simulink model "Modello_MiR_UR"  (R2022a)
settings: Solver=FixedStepAuto  StartTime=0.0  StopTime=time_s(end,1)  FixedStep=Sim.dt*10  RelTol=1e-3  EnableMultiTasking=on
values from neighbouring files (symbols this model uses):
  a = 0.250    (= 0.25)    [Modello_MiR_UR_script.m]    (also in Modello_MiR_2ruote_script.m; Modello_MiR_6ruote_script.m; Modello_MiR_6ruote_validato_script.m)
  a1 = 0.18265    [Modello_MiR_UR_script.m]    (also in UR_DHtable_e.m = 0; Modello_MiR_2ruote_script.m = deg2rad(5); Modello_MiR_6ruote_script.m = deg2rad(5); Modello_MiR_6ruote_validato_script.m)
  a2 = 0.40857    [Modello_MiR_UR_script.m]    (also in UR_DHtable_e.m = 612; Modello_MiR_2ruote_script.m = deg2rad(25); Modello_MiR_6ruote_script.m = deg2rad(25); Modello_MiR_6ruote_validato_script.m)
  Att_C1 = 0.01    [Modello_MiR_UR_script.m]    (also in Modello_MiR_6ruote_validato_script.m)
  Att_C2 = 0.01    [Modello_MiR_UR_script.m]    (also in Modello_MiR_6ruote_validato_script.m)
  Att_C5 = 0.01    [Modello_MiR_UR_script.m]    (also in Modello_MiR_6ruote_validato_script.m)
  Att_C6 = 0.01    [Modello_MiR_UR_script.m]    (also in Modello_MiR_6ruote_validato_script.m)
  b = 0.1875    [Modello_MiR_UR_script.m]    (also in Modello_MiR_2ruote_script.m; Modello_MiR_6ruote_script.m; Modello_MiR_6ruote_validato_script.m)
  b_caster = 0.07    [Modello_MiR_UR_script.m]    (also in Modello_MiR_2ruote_script.m; Modello_MiR_6ruote_script.m; Modello_MiR_6ruote_validato_script.m)
  bd = 0.205    [Modello_MiR_UR_script.m]    (also in Modello_MiR_2ruote_script.m; Modello_MiR_6ruote_script.m; Modello_MiR_6ruote_validato_script.m)
  F23MIR = @(u) (mv*9.801/4)-(mv*h*u(5)+(mv*9.801/4)*(2*a-b_caster*(cos(u(1))+cos(u(2)))))/(4*a-b_caster*(cos(u(1))+cos(u(2)))+b_caster*(cos(u(3))+cos(u(4))))    [Modello_MiR_UR_script.m]
  F23UR5 = @(u) (u(7)/4)-u(11)    [Modello_MiR_UR_script.m]
  F43MIR = @(u) (1/(2*bd))*(mv*u(6)*h+((mv*h*u(5)+(mv*9.801/4)*(2*a-b_caster*(cos(u(1))+cos(u(2)))))/(4*a-b_caster*(cos(u(1))+cos(u(2)))+b_caster*(cos(u(3))+cos(u(4)))))*(2*bd-b_caster*(sin(u(3))+sin(u(4))))+((mv*9.801/4)-(mv*h*u(5)+(mv*9.801/4)*(2*a-b_caster*(cos(u(1))+cos(u(2)))))/(4*a-b_caster*(cos(u(1))+cos(u(2)))+b_caster*(cos(u(3))+cos(u(4)))))*(2*bd-b_caster*(sin(u(1))+sin(u(2)))))    [Modello_MiR_UR_script.m]
  F43UR5 = @(u) (1/(2*bd))*(u(8) - u(6)*H +u(11)*(2*bd-b_caster*(sin(u(3))+sin(u(4))))+u(12)*(2*bd-b_caster*(sin(u(1))+sin(u(2)))))    [Modello_MiR_UR_script.m]
  F63MIR = @(u) (mv*h*u(5)+(mv*9.801/4)*(2*a-b_caster*(cos(u(1))+cos(u(2)))))/(4*a-b_caster*(cos(u(1))+cos(u(2)))+b_caster*(cos(u(3))+cos(u(4))))    [Modello_MiR_UR_script.m]
  F63UR5 = @(u)(-a*u(7)/2 -u(5)*H -u(9) +(u(7)/4)*(2*a-b_caster*(cos(u(1))+cos(u(2)))))/(4*a-b_caster*(cos(u(1))+cos(u(2)))+b_caster*(cos(u(3))+cos(u(4))))    [Modello_MiR_UR_script.m]
  f_c = 0.29564    [Modello_MiR_UR_script.m]    (also in Modello_MiR_6ruote_validato_script.m)
  f_d3 = 0.35846    [Modello_MiR_UR_script.m]    (also in Modello_MiR_6ruote_validato_script.m)
  f_d4 = 0.2333    [Modello_MiR_UR_script.m]    (also in Modello_MiR_6ruote_validato_script.m)
  fa_c = 0.27474    [Modello_MiR_UR_script.m]    (also in Modello_MiR_6ruote_validato_script.m)
  fa_d3 = 0.3694    [Modello_MiR_UR_script.m]    (also in Modello_MiR_6ruote_validato_script.m)
  fa_d4 = 0.28065    [Modello_MiR_UR_script.m]    (also in Modello_MiR_6ruote_validato_script.m)
  fm_fun = @(u) (u <= -am2 || u >= am2) * 0 + (u > -am2 && u <= -am1) * (- u* Mza/(am2 -am1) - Mza* am2/(am2 -am1)) +           + (u > -am1 && u <= am1) * (Mza * u / am1) + (u > am1 && u < am2) * (Mza * u /(am1 -am2) - Mza * am2 /(am1 - am2))    [Modello_MiR_UR_script.m]    (also in Modello_MiR_6ruote_script.m = @(u) (u <= -am2 | u >= am2)*0 + (u > -am2 && u <= -am1)*(- u; Modello_MiR_6ruote_validato_script.m)
  Hi = 1    [UR5e_data.m]
  Icw_1 = 1/2 * mcw * rc^2    (= 0.002004225735)    [Modello_MiR_UR_script.m]    (also in Modello_MiR_2ruote_script.m; Modello_MiR_6ruote_script.m; Modello_MiR_6ruote_validato_script.m)
  Icw_2 = 1/12 * mcw * ec^2 + 1/4 * mcw * rc^2    (= 0.00104098243873)    [Modello_MiR_UR_script.m]    (also in Modello_MiR_2ruote_script.m; Modello_MiR_6ruote_script.m; Modello_MiR_6ruote_validato_script.m)
  Idw_1 = 1/2 * mdw * rd^2    (= 0.00551836278784)    [Modello_MiR_UR_script.m]    (also in Modello_MiR_2ruote_script.m; Transfer_Function_Gol_Gcl.m = Inertia_vect(jj,1); Modello_MiR_6ruote_script.m; Modello_MiR_6ruote_validato_script.m)
  iMax = 20.7*1.1    (= 22.77)    [Modello_MiR_UR_script.m]    (also in Modello_MiR_2ruote_script.m; Modello_MiR_6ruote_script.m; Modello_MiR_6ruote_validato_script.m)
  Iv = mv * (l^2 + w^2)  / 12    (= 6.75343333333)    [Modello_MiR_UR_script.m]    (also in Modello_MiR_2ruote_script.m; Modello_MiR_6ruote_script.m; Modello_MiR_6ruote_validato_script.m = 8.95033333333)
  Kc = 0.15    [Modello_MiR_UR_script.m]    (also in Modello_MiR_2ruote_script.m; Modello_MiR_6ruote_script.m; Modello_MiR_6ruote_validato_script.m)
  Ki_i = 1    [Modello_MiR_UR_script.m]    (also in Modello_MiR_2ruote_script.m; Modello_MiR_6ruote_script.m; Modello_MiR_6ruote_validato_script.m)
  Ki_v = 1    [Modello_MiR_UR_script.m]    (also in Modello_MiR_2ruote_script.m; Modello_MiR_6ruote_script.m; Modello_MiR_6ruote_validato_script.m)
  kk = 0.00005    (= 5e-05)    [Modello_MiR_UR_script.m]    (also in Modello_MiR_2ruote_script.m; Modello_MiR_6ruote_script.m; Modello_MiR_6ruote_validato_script.m)
  Kp_i = 5    [Modello_MiR_UR_script.m]    (also in Modello_MiR_2ruote_script.m; Modello_MiR_6ruote_script.m; Modello_MiR_6ruote_validato_script.m)
  Kp_v = 5    [Modello_MiR_UR_script.m]    (also in Modello_MiR_2ruote_script.m; Modello_MiR_6ruote_script.m; Modello_MiR_6ruote_validato_script.m)
  kv = 1.5e-6    (= 1.5e-06)    [Modello_MiR_UR_script.m]    (also in Modello_MiR_2ruote_script.m; Modello_MiR_6ruote_script.m; Modello_MiR_6ruote_validato_script.m)
  L = R * tauE    (= 0.00181134822805)    [Modello_MiR_UR_script.m]    (also in Modello_MiR_2ruote_script.m; Modello_MiR_6ruote_script.m; Modello_MiR_6ruote_validato_script.m)
  mcw = rc^2 * pi * ec * rhopoliu + 1    (= 1.02616357632)    [Modello_MiR_UR_script.m]    (also in Modello_MiR_2ruote_script.m; Modello_MiR_6ruote_script.m; Modello_MiR_6ruote_validato_script.m)
  mv = 83    [Modello_MiR_UR_script.m]    (also in Modello_MiR_2ruote_script.m; Modello_MiR_6ruote_script.m; Modello_MiR_6ruote_validato_script.m = 110)
  Phi1_start = psi_mir(1,1)    [Modello_MiR_UR_script.m]    (also in Modello_MiR_6ruote_validato_script.m)
  Phi2_start = psi_mir(1,1)    [Modello_MiR_UR_script.m]    (also in Modello_MiR_6ruote_validato_script.m)
  Phi5_start = psi_mir(1,1)    [Modello_MiR_UR_script.m]    (also in Modello_MiR_6ruote_validato_script.m)
  Phi6_start = psi_mir(1,1)    [Modello_MiR_UR_script.m]    (also in Modello_MiR_6ruote_validato_script.m)
  Psi_start = psi_mir(1,1)    [Modello_MiR_UR_script.m]    (also in Modello_MiR_6ruote_script.m = 1.57079632679; Modello_MiR_6ruote_validato_script.m)
  q0 = [qset.q1.signals.values(1),qset.q2.signals.values(1),qset.q3.signals.values(1),qset.q4.signals.values(1),qset.q5.signals.values(1),qset.q6.signals.values(1)]    [UR5e_simmot.m]
  R = velMax * TorqueMax / (iMax)^2    (= 1.81134822805)    [Modello_MiR_UR_script.m]    (also in Modello_MiR_2ruote_script.m; Modello_MiR_6ruote_script.m; Modello_MiR_6ruote_validato_script.m)
  rap_rid = 10.167    [Modello_MiR_UR_script.m]    (also in Modello_MiR_2ruote_script.m; Modello_MiR_6ruote_script.m; Modello_MiR_6ruote_validato_script.m)
  rc = 0.125/2    (= 0.0625)    [Modello_MiR_UR_script.m]    (also in Modello_MiR_2ruote_script.m; Modello_MiR_6ruote_script.m; Modello_MiR_6ruote_validato_script.m)
  rd = 0.1    [Modello_MiR_UR_script.m]    (also in Modello_MiR_2ruote_script.m; Modello_MiR_6ruote_script.m; Modello_MiR_6ruote_validato_script.m)
  s = 1i*s    [Transfer_Function_Gol_Gcl.m]
  s1 = 0.18987    [Modello_MiR_UR_script.m]    (also in Modello_MiR_2ruote_script.m = 0.2; Modello_MiR_6ruote_script.m = 0.2; Modello_MiR_6ruote_validato_script.m)
  s2 = 0.99533    [Modello_MiR_UR_script.m]    (also in Modello_MiR_2ruote_script.m = 0.8; Modello_MiR_6ruote_script.m = 0.8; Modello_MiR_6ruote_validato_script.m)
  Sx = spline(x ,fl_fun(x),zx)    [Modello_MiR_6ruote_script.m]
  Sy = spline(x ,ft_fun(x),zy)    [Modello_MiR_6ruote_script.m]
  tau_i = 1/(2000*2*pi)    (= 7.95774715459e-05)    [UR5e_data.m]    (also in Transfer_Function_Gol_Gcl.m = Kp_i/Ki_i)
  VaMax = Kc * velMax    (= 41.2443991527)    [Modello_MiR_UR_script.m]    (also in Modello_MiR_2ruote_script.m; Modello_MiR_6ruote_script.m; Modello_MiR_6ruote_validato_script.m)
  X_start = traj(1,1)    [Modello_MiR_UR_script.m]    (also in Modello_MiR_2ruote_script.m = input('Inserire coordinata x iniziale'); Modello_MiR_6ruote_script.m = input('Inserire coordinata x iniziale'); Modello_MiR_6ruote_validato_script.m)
  Y_start = traj(1,2)    [Modello_MiR_UR_script.m]    (also in Modello_MiR_2ruote_script.m = input('Inserire coordinata y iniziale'); Modello_MiR_6ruote_script.m = input('Inserire coordinata y iniziale'); Modello_MiR_6ruote_validato_script.m)
undefined symbols (not defined in the file or in its folder): deg, Driver1, Driver2, Driver3, Driver4, Driver5, Driver6, Ground, J1, J2, J3, J4, J5, J6, kg, L1, L2, L3, L4, L5, L6, m, Motor, N, X, Y, z, Z
libraries: sm_lib x33, nesl_utility x30, slpidlib x10
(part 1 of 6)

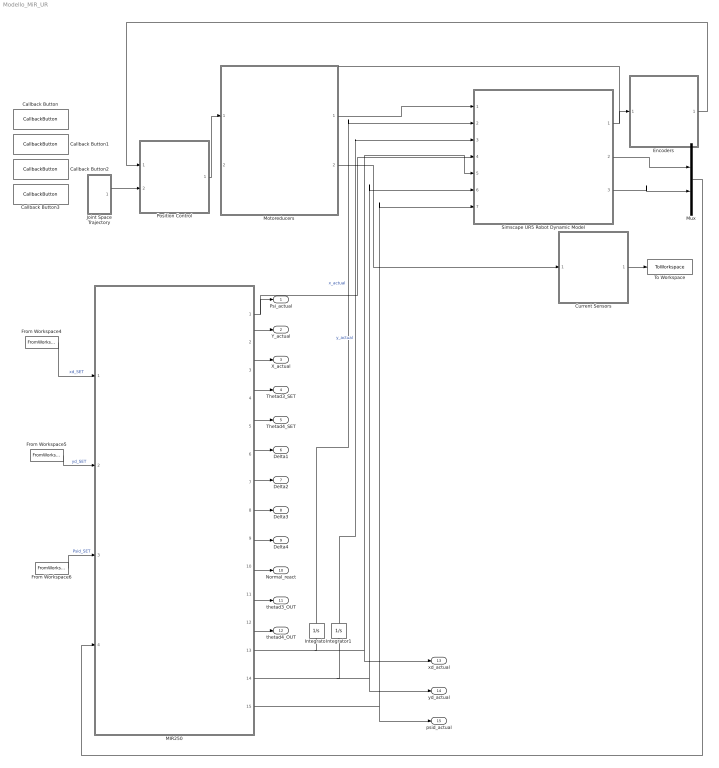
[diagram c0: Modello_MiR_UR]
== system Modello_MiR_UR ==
  Callback Button : CallbackButton  ButtonText=Reset
  Callback Button1 : CallbackButton  ButtonText=Parameters Setting
  Callback Button2 : CallbackButton  ButtonText=Motion Setting
  Callback Button3 : CallbackButton  ButtonText=Current Plotting
  Current Sensors : Subsystem
  Encoders : Subsystem
  From Workspace4 : FromWorkspace  VariableName=[time_v xd_set]
  From Workspace5 : FromWorkspace  VariableName=[time_v yd_set]
  From Workspace6 : FromWorkspace  VariableName=[ time_v psid_set]
  Integrator : Integrator
  Integrator1 : Integrator
  Joint Space Trajectory : Subsystem
  MIR250 : Subsystem
  Motoreducers : Subsystem
  Mux : Mux  Inputs=2
  Position Control : Subsystem
  Simscape UR5 Robot Dynamic Model : Subsystem
  To Workspace : ToWorkspace  VariableName=iFB  SaveFormat=Timeseries  SampleTime=-1
  Psi_actual : Outport
  Y_actual : Outport  Port=2
  X_actual : Outport  Port=3
  Thetad3_SET : Outport  Port=4
  Thetad4_SET : Outport  Port=5
  Delta1 : Outport  Port=6
  Delta2 : Outport  Port=7
  Delta3 : Outport  Port=8
  Delta4 : Outport  Port=9
  Normal_react : Outport  Port=10
  thetad3_OUT : Outport  Port=11
  thetad4_OUT : Outport  Port=12
  xd_actual : Outport  Port=13
  yd_actual : Outport  Port=14
  psid_actual : Outport  Port=15
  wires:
  Encoders/1(qFB,qdFB,qddFB) -> Position Control/1(qFB,qdFB,qddFB)
  Position Control/1(Vset) -> Motoreducers/1(Vset)
  Simscape UR5 Robot Dynamic Model/1(q,qd,qdd) -> Encoders/1(q,qd,qdd), Motoreducers/2(q,qd,qdd)
  Motoreducers/1(Tu) -> Simscape UR5 Robot Dynamic Model/1(T)
  Motoreducers/2(i) -> Current Sensors/1(i)
  Current Sensors/1(iFB) -> To Workspace/1
  Joint Space Trajectory/1(qset) -> Position Control/2(qset,qdset,qddset)
  From Workspace4/1 -> MIR250/1(xd_set)  "xd_SET"
  From Workspace5/1 -> MIR250/2(yd_set)  "yd_SET"
  From Workspace6/1 -> MIR250/3(Psid_set)  "Psid_SET"
  Simscape UR5 Robot Dynamic Model/2(Force constrain) -> Mux/1
  Simscape UR5 Robot Dynamic Model/3(Torque constrain) -> Mux/2
  MIR250/1(Psi_actual) -> Simscape UR5 Robot Dynamic Model/4(psi_actual), Psi_actual/1
  MIR250/2(Y_actual) -> Y_actual/1
  MIR250/3(X_actual) -> X_actual/1
  MIR250/4(Thetad3_SET) -> Thetad3_SET/1
  MIR250/5(Thetad4 SET) -> Thetad4_SET/1
  MIR250/6(Delta1) -> Delta1/1
  MIR250/7(Delta2) -> Delta2/1
  MIR250/8(Delta3) -> Delta3/1
  MIR250/9(Delta4) -> Delta4/1
  MIR250/10(Normal_react) -> Normal_react/1
  MIR250/11(thetad3_OUT) -> thetad3_OUT/1
  MIR250/12(Thetad4_OUT) -> thetad4_OUT/1
  Mux/1 -> MIR250/4(UR5_forces)
  Integrator/1 -> Simscape UR5 Robot Dynamic Model/2(x_actual)  "x_actual"
  Integrator1/1 -> Simscape UR5 Robot Dynamic Model/3(y_actual)  "y_actual"
  MIR250/13(xd_actual) -> xd_actual/1, Simscape UR5 Robot Dynamic Model/5(xd_actual), Integrator/1
  MIR250/14(yd_actual) -> Simscape UR5 Robot Dynamic Model/6(yd_actual), yd_actual/1, Integrator1/1
  MIR250/15(Psid_actual) -> psid_actual/1, Simscape UR5 Robot Dynamic Model/7(psid_actual)

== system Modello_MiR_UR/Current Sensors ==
  i : Inport
  Demux1 : Demux  Outputs=6
  Mux1 : Mux  Inputs=6
  Subsystem : Subsystem
  iFB : Outport
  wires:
  Subsystem/1(i1FB) -> Mux1/1
  Demux1/4 -> Subsystem/4(i5)
  Demux1/5 -> Subsystem/5(i3)
  Subsystem/6(i6FB) -> Mux1/6
  Demux1/2 -> Subsystem/2(i4)
  Subsystem/3(i2FB) -> Mux1/3
  Demux1/6 -> Subsystem/6(i6)
  Demux1/3 -> Subsystem/3(i2)
  Demux1/1 -> Subsystem/1(i1)
  Subsystem/4(i5FB) -> Mux1/4
  Subsystem/2(i4FB) -> Mux1/2
  Subsystem/5(i3FB) -> Mux1/5
  Mux1/1 -> iFB/1
  i/1 -> Demux1/1

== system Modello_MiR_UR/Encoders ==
  q,qd,qdd : Inport
  Demux1 : Demux  Outputs=6
  Mux1 : Mux  Inputs=6
  Subsystem : Subsystem
  qFB,qdFB,qddFB : Outport
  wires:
  q,qd,qdd/1 -> Demux1/1
  Mux1/1 -> qFB,qdFB,qddFB/1
  Subsystem/5(q5FB,qd5FB,qdd5FB) -> Mux1/5
  Subsystem/2(q2FB,qd2FB,qdd2FB) -> Mux1/2
  Subsystem/4(q4FB,qd4FB,qdd4FB) -> Mux1/4
  Demux1/1 -> Subsystem/1(q1,qd1,qdd2)
  Demux1/3 -> Subsystem/3(q3,qd3,qdd3)
  Demux1/6 -> Subsystem/6(q6,qd6,qdd6)
  Subsystem/3(q3FB,qd3FB,qdd3FB) -> Mux1/3
  Demux1/2 -> Subsystem/2(q2,qd2,qdd2)
  Subsystem/6(q6FB,qd6FB,qdd6FB) -> Mux1/6
  Demux1/5 -> Subsystem/5(q5,qd5,qdd5)
  Demux1/4 -> Subsystem/4(q4,qd4,qdd4)
  Subsystem/1(q1FB,qd1FB,qdd1FB) -> Mux1/1

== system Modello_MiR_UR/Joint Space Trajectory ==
  From Workspace : FromWorkspace  VariableName=qset.q1
  From Workspace1 : FromWorkspace  VariableName=qset.q2
  From Workspace2 : FromWorkspace  VariableName=qset.q3
  From Workspace3 : FromWorkspace  VariableName=qset.q4
  From Workspace4 : FromWorkspace  VariableName=qset.q5
  From Workspace5 : FromWorkspace  VariableName=qset.q6
  Mux2 : Mux  Inputs=6
  qset : Outport
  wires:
  From Workspace2/1 -> Mux2/3
  From Workspace/1 -> Mux2/1
  From Workspace3/1 -> Mux2/4
  From Workspace4/1 -> Mux2/5
  From Workspace5/1 -> Mux2/6
  From Workspace1/1 -> Mux2/2
  Mux2/1 -> qset/1

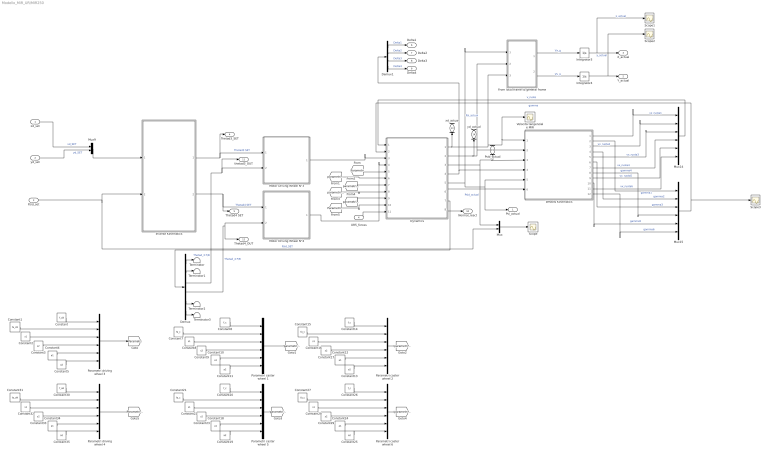
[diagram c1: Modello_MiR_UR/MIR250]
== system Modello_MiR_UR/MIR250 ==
  xd_set : Inport
  yd_set : Inport  Port=2
  Psid_set : Inport  Port=3
  UR5_forces : Inport  Port=4
  " Wheels Kinematics" : Subsystem
  Constant : Constant  Value=f_d3
  Constant1 : Constant  Value=fa_d3
  Constant{4,10,12,18,24,34} (6 alike) : Constant  Value=a1
  Constant{5,11,13,19,25,35} (6 alike) : Constant  Value=a2
  Constant{6,14,20,26} (4 alike) : Constant  Value=f_c
  Constant{7,15,21,27} (4 alike) : Constant  Value=fa_c
  Constant{2,8,16,22,28,32} (6 alike) : Constant  Value=s1
  Constant{3,9,17,23,29,33} (6 alike) : Constant  Value=s2
  Constant30 : Constant  Value=f_d4
  Constant31 : Constant  Value=fa_d4
  Demux : Demux  Outputs=6
  Demux1 : Demux
  Dynamics : Subsystem
  From local frame to general frame : Subsystem
  Integrator3 : Integrator  InitialCondition=X_start
  Integrator4 : Integrator  InitialCondition=Y_start
  Inverse Kinematics : Subsystem
  Motor Driving Wheel N°3 : Subsystem
  Motor Driving Wheel N°4 : Subsystem
  Mux : Mux  Inputs=2
  Mux14 : Mux  Inputs=6
  Mux15 : Mux  Inputs=6
  Mux9 : Mux  Inputs=2
  Parametri caster wheel {1..2,5..6} (4 alike) : Mux  Inputs=6
  Parametri driving wheel 3 : Mux  Inputs=6
  Parametri driving wheel 4 : Mux  Inputs=6
  Scope{,1..3} (4 alike) : Scope
  Terminator{,1..3} (4 alike) : Terminator
  Velocità tangenziale MIR : Scope
  Psi_actual : Outport
  Y_actual : Outport  Port=2
  X_actual : Outport  Port=3
  Thetad3_SET : Outport  Port=4
  Thetad4 SET : Outport  Port=5
  Delta1 : Outport  Port=6
  Delta2 : Outport  Port=7
  Delta3 : Outport  Port=8
  Delta4 : Outport  Port=9
  Normal_react : Outport  Port=10
  thetad3_OUT : Outport  Port=11
  Thetad4_OUT : Outport  Port=12
  xd_actual : Outport  Port=13
  yd_actual : Outport  Port=14
  Psid_actual : Outport  Port=15
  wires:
  Demux1/4 -> Delta4/1  "Delta4"
  Constant5/1 -> Parametri driving wheel 3/6
  [Parametri] -> Dynamics/5(parametri_dw3)
  Demux1/1 -> Delta1/1  "Delta1"
  Mux/1 -> Scope/1
  Motor Driving Wheel N°4/1(Cm_R) -> Dynamics/4(Cm4)
  " Wheels Kinematics"/1(vx_ruota1) -> Mux14/1  "vx_ruota1"
  Mux14/1 -> Dynamics/1(vx_ruote)  "v_ruote"
  From local frame to general frame/1(Vx_g) -> Integrator3/1  "Vx_g"
  Dynamics/2(yd) -> yd_actual/1, From local frame to general frame/2(Vy), " Wheels Kinematics"/2(yd)
  Demux/2 -> Terminator1/1
  Demux/4 -> Thetad4_OUT/1, Motor Driving Wheel N°4/2(ThetadR_FB)  "Thetad_4 F/B"
  Integrator3/1 -> Scope1/1, X_actual/1  "x_actual"
  " Wheels Kinematics"/6(gamma3) -> Mux15/3  "gamma3"
  Mux9/1 -> Inverse Kinematics/1(vSet)
  Integrator4/1 -> Scope2/1, Y_actual/1  "y_actual"
  Dynamics/3(Psid) -> Psid_actual/1, " Wheels Kinematics"/3(Psid), Mux/1  "Psid_actual"
  Demux/5 -> Terminator2/1
  " Wheels Kinematics"/5(vx_ruota3) -> Mux14/3  "vx_ruota3"
  Dynamics/7(Thetad) -> Demux/1
  Demux/6 -> Terminator3/1
  Dynamics/5(Psi) -> From local frame to general frame/1(Psi), Psi_actual/1, " Wheels Kinematics"/5(Psi)  "Psi_actual"
  " Wheels Kinematics"/3(vx_ruota2) -> Mux14/2  "vx_ruota2"
  " Wheels Kinematics"/8(gamma4) -> Mux15/4  "gamma4"
  " Wheels Kinematics"/7(vx_ruota4) -> Mux14/4  "vx_ruota4"
  Dynamics/4(Delta) -> Demux1/1, " Wheels Kinematics"/4(Delta)
  From local frame to general frame/2(Vy_g) -> Integrator4/1  "Vy_g"
  " Wheels Kinematics"/12(gamma6) -> Mux15/6  "gamma6"
  " Wheels Kinematics"/4(gamma2) -> Mux15/2  "gamma2"
  Constant20/1 -> Parametri caster wheel 5/1
  Parametri caster wheel 6/1 -> [parametri_cw6]
  yd_set/1 -> Mux9/2  "yd_SET"
  Demux1/2 -> Delta2/1  "Delta2"
  Constant27/1 -> Parametri caster wheel 6/2
  Constant21/1 -> Parametri caster wheel 5/2
  [parametri_cw5] -> Dynamics/8(parametri_cw5)
  " Wheels Kinematics"/9(vx_ruota5) -> Mux14/5  "vx_ruota5"
  Constant26/1 -> Parametri caster wheel 6/1
  Constant24/1 -> Parametri caster wheel 6/5
  Motor Driving Wheel N°3/1(Cm_L) -> Dynamics/3(Cm3)
  [parametri_cw2] -> Dynamics/7(parametri_cw2)
  Constant28/1 -> Parametri caster wheel 6/3
  Parametri caster wheel 1/1 -> [parametri_cw1]
  Constant29/1 -> Parametri caster wheel 6/4
  Constant6/1 -> Parametri caster wheel 1/1
  Inverse Kinematics/2(ThetaDotR) -> Thetad4 SET/1, Motor Driving Wheel N°4/1(ThetadR_SET)  "Thetad4 SET"
  Constant15/1 -> Parametri caster wheel 2/2
  Parametri driving wheel 3/1 -> [Parametri]
  Constant4/1 -> Parametri driving wheel 3/5
  Parametri caster wheel 2/1 -> [parametri_cw2]
  Constant12/1 -> Parametri caster wheel 2/5
  Constant7/1 -> Parametri caster wheel 1/2
  Dynamics/6(Phid) -> " Wheels Kinematics"/6(Phid)
  Psid_set/1 -> Mux/2, Inverse Kinematics/2(psiDotSet)  "Psid_SET"
  xd_set/1 -> Mux9/1  "xd_SET"
  Constant10/1 -> Parametri caster wheel 1/5
  Mux15/1 -> Scope3/1, Dynamics/2(gamma)  "gamma"
  Constant2/1 -> Parametri driving wheel 3/3
  Constant1/1 -> Parametri driving wheel 3/2
  Dynamics/8(Normal_react) -> Normal_react/1
  Demux/1 -> Terminator/1
  Constant18/1 -> Parametri caster wheel 5/5
  " Wheels Kinematics"/2(gamma1) -> Mux15/1  "gamma1"
  Constant8/1 -> Parametri caster wheel 1/3
  Inverse Kinematics/1(ThetaDotL) -> Thetad3_SET/1, Motor Driving Wheel N°3/1(ThetadL_SET)  "Thetad3 SET"
  Constant17/1 -> Parametri caster wheel 2/4
  Constant16/1 -> Parametri caster wheel 2/3
  Constant30/1 -> Parametri driving wheel 4/1
  Parametri driving wheel 4/1 -> [Parametri_dw4]
  Demux/3 -> thetad3_OUT/1, Motor Driving Wheel N°3/2(ThetadL_FB)  "Thetad_3 F/B"
  [Parametri_dw4] -> Dynamics/10(parametri_dw4)
  Constant3/1 -> Parametri driving wheel 3/4
  Constant22/1 -> Parametri caster wheel 5/3
  " Wheels Kinematics"/11(vx_ruota6) -> Mux14/6  "vx_ruota6"
  " Wheels Kinematics"/10(gamma5) -> Mux15/5  "gamma5"
  Constant34/1 -> Parametri driving wheel 4/5
  Constant31/1 -> Parametri driving wheel 4/2
  Constant9/1 -> Parametri caster wheel 1/4
  Constant32/1 -> Parametri driving wheel 4/3
  Constant11/1 -> Parametri caster wheel 1/6
  [parametri_cw1] -> Dynamics/6(parametri_cw1)
  Dynamics/1(xd) -> xd_actual/1, From local frame to general frame/3(Vx), Velocità tangenziale MIR/1, " Wheels Kinematics"/1(xd)
  Parametri caster wheel 5/1 -> [parametri_cw5]
  Demux1/3 -> Delta3/1  "Delta3"
  Constant33/1 -> Parametri driving wheel 4/4
  Constant14/1 -> Parametri caster wheel 2/1
  Constant19/1 -> Parametri caster wheel 5/6
  Constant13/1 -> Parametri caster wheel 2/6
  [parametri_cw6] -> Dynamics/9(parametri_cw6)
  Constant25/1 -> Parametri caster wheel 6/6
  Constant23/1 -> Parametri caster wheel 5/4
  Constant35/1 -> Parametri driving wheel 4/6
  Constant/1 -> Parametri driving wheel 3/1
  UR5_forces/1 -> Dynamics/11(UR5_forces)

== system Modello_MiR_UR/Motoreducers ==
  Vset : Inport
  q,qd,qdd : Inport  Port=2
  Demux1 : Demux  Outputs=6
  Demux2 : Demux  Outputs=6
  Mux1 : Mux  Inputs=6
  Mux2 : Mux  Inputs=6
  Subsystem : Subsystem
  Tu : Outport
  i : Outport  Port=2
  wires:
  Vset/1 -> Demux1/1
  Mux1/1 -> Tu/1
  Subsystem/5(Tu5) -> Mux1/5
  Subsystem/2(Tu2) -> Mux1/2
  Subsystem/4(Tu4) -> Mux1/4
  Demux1/1 -> Subsystem/1(Vset1)
  Demux1/3 -> Subsystem/3(Vset3)
  Demux1/6 -> Subsystem/6(Vset6)
  Subsystem/3(Tu3) -> Mux1/3
  Demux1/2 -> Subsystem/2(Vset2)
  Subsystem/6(Tu6) -> Mux1/6
  Demux1/5 -> Subsystem/5(Vset5)
  Demux1/4 -> Subsystem/4(Vset4)
  Subsystem/1(Tu1) -> Mux1/1
  Demux2/1 -> Subsystem/7(q1,qd1,qdd1)
  Demux2/2 -> Subsystem/8(q2,qd2,qdd2)
  Demux2/3 -> Subsystem/9(q3,qd3,qdd3)
  Demux2/4 -> Subsystem/10(q4,qd4,qdd4)
  Demux2/5 -> Subsystem/11(q5,qd5,qdd5)
  Demux2/6 -> Subsystem/12(q6,qd6,qdd6)
  q,qd,qdd/1 -> Demux2/1
  Subsystem/7(i1) -> Mux2/1
  Subsystem/8(i2) -> Mux2/2
  Subsystem/9(i3) -> Mux2/3
  Subsystem/10(i4) -> Mux2/4
  Subsystem/11(i5) -> Mux2/5
  Subsystem/12(i6) -> Mux2/6
  Mux2/1 -> i/1

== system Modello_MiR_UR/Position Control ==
  qFB,qdFB,qddFB : Inport
  qset,qdset,qddset : Inport  Port=2
  Demux : Demux  Outputs=6
  Demux1 : Demux  Outputs=6
  Mux : Mux  Inputs=6
  Subsystem : Subsystem
  Vset : Outport
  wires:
  Demux/1 -> Subsystem/1(q1set,qd1set,qdd1set)
  Demux/4 -> Subsystem/4(q4set,qd4set,qdd4set)
  Demux/3 -> Subsystem/3(q3set,qd3set,qdd3set)
  Demux1/1 -> Subsystem/7(q1FB,qd1FB,qdd1FB)
  Demux/5 -> Subsystem/5(q5set,qd5set,qdd5set)
  Demux1/2 -> Subsystem/8(q2FB,qd2FB,qdd2FB)
  Demux/2 -> Subsystem/2(q2set,qd2set,qdd2set)
  Demux/6 -> Subsystem/6(q6set,qd6set,qdd6set)
  Demux1/3 -> Subsystem/9(q3FB,qd3FB,qdd3FB)
  Demux1/5 -> Subsystem/11(q5FB,qd5FB,qdd5FB)
  Demux1/6 -> Subsystem/12(q6FB,qd6FB,qdd6FB)
  Subsystem/4(Vset4) -> Mux/4
  Demux1/4 -> Subsystem/10(q4FB,qd4FB,qdd4FB)
  Subsystem/2(Vset2) -> Mux/2
  Subsystem/1(Vset1) -> Mux/1
  Subsystem/5(Vset5) -> Mux/5
  Subsystem/6(Vset6) -> Mux/6
  Subsystem/3(Vset3) -> Mux/3
  qFB,qdFB,qddFB/1 -> Demux1/1
  Mux/1 -> Vset/1
  qset,qdset,qddset/1 -> Demux/1

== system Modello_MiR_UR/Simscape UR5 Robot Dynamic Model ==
  T : Inport
  x_actual : Inport  Port=2
  y_actual : Inport  Port=3
  psi_actual : Inport  Port=4
  xd_actual : Inport  Port=5
  yd_actual : Inport  Port=6
  psid_actual : Inport  Port=7
  Demux1 : Demux  Outputs=6
  Mux1 : Mux  Inputs=6
  Sinscape UR5 Robot Dynamic Model1 : Subsystem
  q,qd,qdd : Outport
  Force constrain : Outport  Port=2
  Torque constrain : Outport  Port=3
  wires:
  Sinscape UR5 Robot Dynamic Model1/1(q1,qd1,qdd1) -> Mux1/1
  Demux1/4 -> Sinscape UR5 Robot Dynamic Model1/4(T4)
  Demux1/5 -> Sinscape UR5 Robot Dynamic Model1/5(T5)
  Sinscape UR5 Robot Dynamic Model1/6(q6,qd6,qdd6) -> Mux1/6
  Demux1/2 -> Sinscape UR5 Robot Dynamic Model1/2(T2)
  Sinscape UR5 Robot Dynamic Model1/3(q3,qd3,qdd3) -> Mux1/3
  Demux1/6 -> Sinscape UR5 Robot Dynamic Model1/6(T6)
  Demux1/3 -> Sinscape UR5 Robot Dynamic Model1/3(T3)
  Demux1/1 -> Sinscape UR5 Robot Dynamic Model1/1(T1)
  Sinscape UR5 Robot Dynamic Model1/4(q4,qd4,qdd4) -> Mux1/4
  Sinscape UR5 Robot Dynamic Model1/2(q2,qd2,qdd2) -> Mux1/2
  Sinscape UR5 Robot Dynamic Model1/5(q5,qd5,qdd5) -> Mux1/5
  Mux1/1 -> q,qd,qdd/1
  T/1 -> Demux1/1
  x_actual/1 -> Sinscape UR5 Robot Dynamic Model1/7(x_actual)
  y_actual/1 -> Sinscape UR5 Robot Dynamic Model1/8(y_actual)
  psi_actual/1 -> Sinscape UR5 Robot Dynamic Model1/9(psi_actual)
  Sinscape UR5 Robot Dynamic Model1/7(Force constrain) -> Force constrain/1
  Sinscape UR5 Robot Dynamic Model1/8(Torque constrain) -> Torque constrain/1
  xd_actual/1 -> Sinscape UR5 Robot Dynamic Model1/10(xd_actual)
  yd_actual/1 -> Sinscape UR5 Robot Dynamic Model1/11(yd_actual)
  psid_actual/1 -> Sinscape UR5 Robot Dynamic Model1/12(psid_actual)

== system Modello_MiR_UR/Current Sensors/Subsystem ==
  i1 : Inport
  i4 : Inport  Port=2
  i2 : Inport  Port=3
  i5 : Inport  Port=4
  i3 : Inport  Port=5
  i6 : Inport  Port=6
  Current Sensor{1..6} (6 alike) : TransferFcn  Numerator=[Hi]  Denominator=[tau_i 1]
  i1FB : Outport
  i4FB : Outport  Port=2
  i2FB : Outport  Port=3
  i5FB : Outport  Port=4
  i3FB : Outport  Port=5
  i6FB : Outport  Port=6
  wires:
  i6/1 -> Current Sensor6/1
  i2/1 -> Current Sensor2/1
  Current Sensor2/1 -> i2FB/1
  i1/1 -> Current Sensor1/1
  Current Sensor3/1 -> i3FB/1
  Current Sensor6/1 -> i6FB/1
  i3/1 -> Current Sensor3/1
  i4/1 -> Current Sensor4/1
  Current Sensor1/1 -> i1FB/1
  Current Sensor4/1 -> i4FB/1
  i5/1 -> Current Sensor5/1
  Current Sensor5/1 -> i5FB/1

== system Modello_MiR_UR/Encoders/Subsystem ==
  q1,qd1,qdd2 : Inport
  q2,qd2,qdd2 : Inport  Port=2
  q3,qd3,qdd3 : Inport  Port=3
  q4,qd4,qdd4 : Inport  Port=4
  q5,qd5,qdd5 : Inport  Port=5
  q6,qd6,qdd6 : Inport  Port=6
  Gain{,1..5} (6 alike) : Gain
  q1FB,qd1FB,qdd1FB : Outport
  q2FB,qd2FB,qdd2FB : Outport  Port=2
  q3FB,qd3FB,qdd3FB : Outport  Port=3
  q4FB,qd4FB,qdd4FB : Outport  Port=4
  q5FB,qd5FB,qdd5FB : Outport  Port=5
  q6FB,qd6FB,qdd6FB : Outport  Port=6
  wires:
  q2,qd2,qdd2/1 -> Gain1/1
  Gain3/1 -> q4FB,qd4FB,qdd4FB/1
  Gain/1 -> q1FB,qd1FB,qdd1FB/1
  Gain1/1 -> q2FB,qd2FB,qdd2FB/1
  q4,qd4,qdd4/1 -> Gain3/1
  q3,qd3,qdd3/1 -> Gain2/1
  Gain5/1 -> q6FB,qd6FB,qdd6FB/1
  Gain2/1 -> q3FB,qd3FB,qdd3FB/1
  Gain4/1 -> q5FB,qd5FB,qdd5FB/1
  q1,qd1,qdd2/1 -> Gain/1
  q5,qd5,qdd5/1 -> Gain4/1
  q6,qd6,qdd6/1 -> Gain5/1

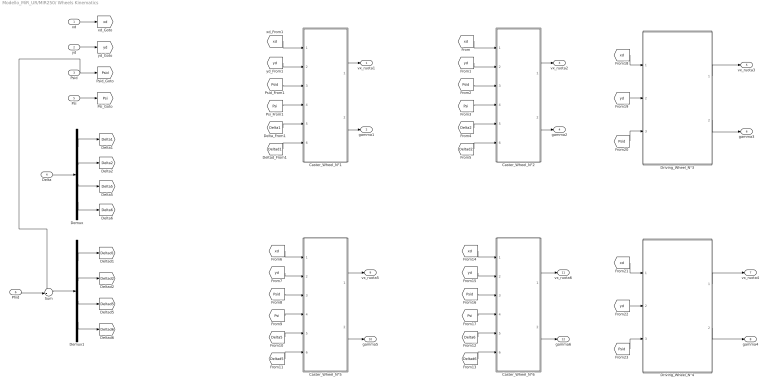
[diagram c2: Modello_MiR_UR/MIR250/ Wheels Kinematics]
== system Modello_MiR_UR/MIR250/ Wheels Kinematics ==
  xd : Inport
  yd : Inport  Port=2
  Psid : Inport  Port=3
  Delta : Inport  Port=4
  Psi : Inport  Port=5
  Phid : Inport  Port=6
  Caster_Wheel_N°1 : Subsystem
  Caster_Wheel_N°2 : Subsystem
  Caster_Wheel_N°5 : Subsystem
  Caster_Wheel_N°6 : Subsystem
  Demux : Demux
  Demux1 : Demux
  Driving_Wheel_N°3 : Subsystem
  Driving_Wheel_N°4 : Subsystem
  Sum : Sum  Inputs=-+|
  vx_ruota1 : Outport
  gamma1 : Outport  Port=2  PortDimensions=1
  vx_ruota2 : Outport  Port=3
  gamma2 : Outport  Port=4  PortDimensions=1
  vx_ruota3 : Outport  Port=5
  gamma3 : Outport  Port=6  PortDimensions=1
  vx_ruota4 : Outport  Port=7
  gamma4 : Outport  Port=8  PortDimensions=1
  vx_ruota5 : Outport  Port=9
  gamma5 : Outport  Port=10  PortDimensions=1
  vx_ruota6 : Outport  Port=11
  gamma6 : Outport  Port=12  PortDimensions=1
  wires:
  xd/1 -> [xd]
  yd/1 -> [yd]
  Psid/1 -> [Psid], Sum/1
  Delta/1 -> Demux/1
  Demux/1 -> [Delta1]
  Demux/2 -> [Delta2]
  Demux/3 -> [Delta5]
  Demux/4 -> [Delta6]
  Psi/1 -> [Psi]
  Phid/1 -> Sum/2
  Demux1/1 -> [Deltad1]
  Demux1/2 -> [Deltad2]
  Demux1/3 -> [Deltad5]
  Demux1/4 -> [Deltad6]
  [xd] -> Caster_Wheel_N°1/1(xd_From1)
  [yd] -> Caster_Wheel_N°1/2(yd_From1)
  [Psid] -> Caster_Wheel_N°1/3(Psid_From1)
  [Psi] -> Caster_Wheel_N°1/4(Psi_From1)
  [Delta1] -> Caster_Wheel_N°1/5(Delta_From1)
  [Deltad1] -> Caster_Wheel_N°1/6(Deltad_From1)
  Caster_Wheel_N°1/1(vx_ruota1) -> vx_ruota1/1
  Caster_Wheel_N°1/2(gamma1) -> gamma1/1
  [yd] -> Caster_Wheel_N°2/2(yd_From1)
  [Psi] -> Caster_Wheel_N°2/4(Psi_From1)
  [Psid] -> Caster_Wheel_N°2/3(Psid_From1)
  [xd] -> Caster_Wheel_N°2/1(xd_From1)
  [Deltad2] -> Caster_Wheel_N°2/6(Deltad_From2)
  Caster_Wheel_N°2/2(gamma2) -> gamma2/1
  [Delta2] -> Caster_Wheel_N°2/5(Delta_From2)
  Caster_Wheel_N°2/1(vx_ruota2) -> vx_ruota2/1
  [xd] -> Caster_Wheel_N°5/1(xd_From1)
  Caster_Wheel_N°5/2(gamma5) -> gamma5/1
  Caster_Wheel_N°5/1(vx_ruota5) -> vx_ruota5/1
  [Psid] -> Caster_Wheel_N°5/3(Psid_From1)
  [Deltad5] -> Caster_Wheel_N°5/6(Deltad_From5)
  [yd] -> Caster_Wheel_N°5/2(yd_From1)
  [Delta5] -> Caster_Wheel_N°5/5(Delta_From5)
  [Psi] -> Caster_Wheel_N°5/4(Psi_From1)
  Caster_Wheel_N°6/1(vx_ruota6) -> vx_ruota6/1
  [yd] -> Caster_Wheel_N°6/2(yd_From1)
  [Psid] -> Caster_Wheel_N°6/3(Psid_From1)
  [Psi] -> Caster_Wheel_N°6/4(Psi_From1)
  Caster_Wheel_N°6/2(gamma6) -> gamma6/1
  [xd] -> Caster_Wheel_N°6/1(xd_From1)
  [Delta6] -> Caster_Wheel_N°6/5(Delta_From6)
  [Deltad6] -> Caster_Wheel_N°6/6(Deltad_From6)
  [xd] -> Driving_Wheel_N°3/1(xd_From1)
  [yd] -> Driving_Wheel_N°3/2(yd_From1)
  [Psid] -> Driving_Wheel_N°3/3(Psid_From1)
  [xd] -> Driving_Wheel_N°4/1(xd_From1)
  [yd] -> Driving_Wheel_N°4/2(yd_From1)
  [Psid] -> Driving_Wheel_N°4/3(Psid_From1)
  Driving_Wheel_N°3/1(vx_ruota3) -> vx_ruota3/1
  Driving_Wheel_N°3/2(gamma3) -> gamma3/1
  Driving_Wheel_N°4/1(vx_ruota4) -> vx_ruota4/1
  Driving_Wheel_N°4/2(gamma4) -> gamma4/1
  Sum/1 -> Demux1/1

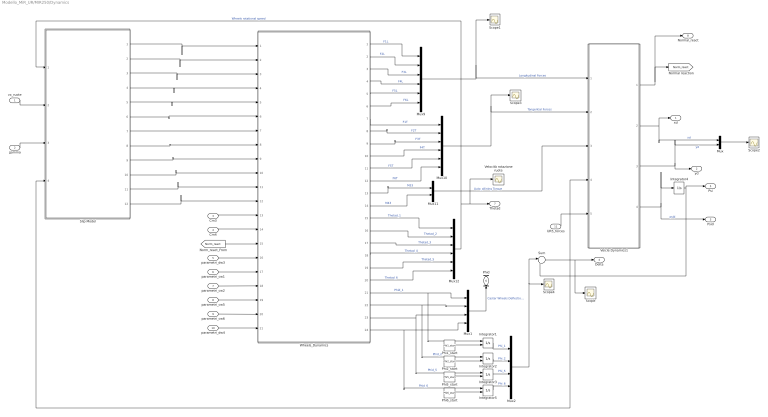
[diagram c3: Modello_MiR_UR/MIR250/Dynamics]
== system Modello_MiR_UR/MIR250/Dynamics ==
  vx_ruote : Inport
  gamma : Inport  Port=2
  Cm3 : Inport  Port=3
  Cm4 : Inport  Port=4
  parametri_dw3 : Inport  Port=5
  parametri_cw1 : Inport  Port=6
  parametri_cw2 : Inport  Port=7
  parametri_cw5 : Inport  Port=8
  parametri_cw6 : Inport  Port=9
  parametri_dw4 : Inport  Port=10
  UR5_forces : Inport  Port=11
  Integrator{1..3,5} (4 alike) : Integrator  InitialConditionSource=external
  Integrator4 : Integrator  InitialCondition=Psi_start
  Mux : Mux  Inputs=2
  Mux1 : Mux
  Mux10 : Mux  Inputs=6
  Mux11 : Mux  Inputs=2
  Mux12 : Mux  Inputs=6
  Mux2 : Mux
  Mux9 : Mux  Inputs=6
  Phi1_start : Constant  Value=Phi1_start
  Phi2_start : Constant  Value=Phi2_start
  Phi5_start : Constant  Value=Phi5_start
  Phi6_start : Constant  Value=Phi6_start
  Scope{,1..4} (5 alike) : Scope
  Slip Model : Subsystem
  Sum : Sum  Inputs=|+-
  Veicle Dynamics1 : Subsystem
  Velocità rotazione ruote : Scope
  Wheels_Dynamics : Subsystem
  xd : Outport
  yd : Outport  Port=2
  Psid : Outport  Port=3
  Delta : Outport  Port=4
  Psi : Outport  Port=5
  Phid : Outport  Port=6
  Thetad : Outport  Port=7
  Normal_react : Outport  Port=8
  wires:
  Wheels_Dynamics/14(M43) -> Mux11/2  "M43"
  Wheels_Dynamics/23(Phid_5) -> Integrator3/1, Mux1/3  "Phid_5"
  Wheels_Dynamics/8(F2T) -> Mux10/2  "F2T"
  Wheels_Dynamics/12(F6T) -> Mux10/6  "F6T"
  Wheels_Dynamics/19(Thetad_5) -> Mux12/5  "Thetad_5"
  Wheels_Dynamics/18(Thetad_4) -> Mux12/4  "Thetad_4"
  Slip Model/1(Sigma1) -> Wheels_Dynamics/1(Sigma1)
  Wheels_Dynamics/2(F2L) -> Mux9/2  "F2L"
  Wheels_Dynamics/4(F4L) -> Mux9/4  "F4L"
  Wheels_Dynamics/3(F3L) -> Mux9/3  "F3L"
  Wheels_Dynamics/1(F1L) -> Mux9/1  "F1L"
  Slip Model/3(Sigma3) -> Wheels_Dynamics/3(Sigma3)
  Slip Model/11(alpha5) -> Wheels_Dynamics/11(alpha5)
  Wheels_Dynamics/5(F5L) -> Mux9/5  "F5L"
  Slip Model/9(alpha3) -> Wheels_Dynamics/9(alpha3)
  Wheels_Dynamics/16(Thetad_2) -> Mux12/2  "Thetad_2"
  Mux1/1 -> Phid/1  "Caster Wheels Deflection Velocity"
  Cm3/1 -> Wheels_Dynamics/13(Cm3)
  Mux11/1 -> Veicle Dynamics1/3(M)  "Auto_allining Torque"
  Wheels_Dynamics/10(F4T) -> Mux10/4  "F4T"
  Wheels_Dynamics/13(M33) -> Mux11/1  "M33"
  Mux12/1 -> Slip Model/1(Thetad_ruote), Velocità rotazione ruote/1, Thetad/1  "Wheels rotational speed"
  Mux10/1 -> Scope3/1, Veicle Dynamics1/2(FT)  "Tangential Forces"
  Slip Model/5(Sigma5) -> Wheels_Dynamics/5(Sigma5)
  Wheels_Dynamics/21(Phid_1) -> Integrator1/1, Mux1/1  "Phid_1"
  Wheels_Dynamics/6(F6L) -> Mux9/6  "F6L"
  Wheels_Dynamics/17(Thetad_3) -> Mux12/3  "Thetad_3"
  Wheels_Dynamics/15(Thetad_1) -> Mux12/1  "Thetad_1"
  Wheels_Dynamics/24(Phid_6) -> Integrator5/1, Mux1/4  "Phid_6"
  Wheels_Dynamics/11(F5T) -> Mux10/5  "F5T"
  Wheels_Dynamics/9(F3T) -> Mux10/3  "F3T"
  Wheels_Dynamics/7(F1T) -> Mux10/1  "F1T"
  Wheels_Dynamics/22(Phid_2) -> Integrator2/1, Mux1/2  "Phid_2"
  Mux2/1 -> Sum/1, Scope4/1
  Wheels_Dynamics/20(Thetad_6) -> Mux12/6  "Thetad_6"
  Slip Model/8(alpha2) -> Wheels_Dynamics/8(alpha2)
  Integrator4/1 -> Psi/1, Sum/2
  [Norm_react] -> Wheels_Dynamics/15(Normal_React)
  Veicle Dynamics1/4(Psid) -> Integrator4/1, Psid/1  "psid"
  Mux9/1 -> Scope1/1, Veicle Dynamics1/1(FL)  "Longitudinal Forces"
  Slip Model/4(Sigma4) -> Wheels_Dynamics/4(Sigma4)
  Slip Model/10(alpha4) -> Wheels_Dynamics/10(alpha4)
  Slip Model/12(alpha6) -> Wheels_Dynamics/12(alpha6)
  Slip Model/7(alpha1) -> Wheels_Dynamics/7(alpha1)
  Slip Model/2(Sigma2) -> Wheels_Dynamics/2(Sigma2)
  Slip Model/6(Sigma6) -> Wheels_Dynamics/6(Sigma6)
  vx_ruote/1 -> Slip Model/2(vx_ruote)
  gamma/1 -> Slip Model/3(gamma)
  Cm4/1 -> Wheels_Dynamics/14(Cm4)
  Mux/1 -> Scope2/1
  Sum/1 -> Veicle Dynamics1/4(Delta), Slip Model/4(Delta), Scope/1, Delta/1
  parametri_dw3/1 -> Wheels_Dynamics/16(parametri_dw3)
  parametri_cw1/1 -> Wheels_Dynamics/17(parametri_cw1)
  parametri_cw2/1 -> Wheels_Dynamics/18(parametri_cw2)
  parametri_cw5/1 -> Wheels_Dynamics/19(parametri_cw5)
  parametri_cw6/1 -> Wheels_Dynamics/20(parametri_cw6)
  Integrator1/1 -> Mux2/1  "Phi_1"
  Integrator2/1 -> Mux2/2  "Phi_2"
  Integrator3/1 -> Mux2/3  "Phi_5"
  Integrator5/1 -> Mux2/4  "Phi_6"
  Phi1_start/1 -> Integrator1/2
  Phi2_start/1 -> Integrator2/2
  Phi5_start/1 -> Integrator3/2
  Phi6_start/1 -> Integrator5/2
  parametri_dw4/1 -> Wheels_Dynamics/21(parametri_dw4)
  Veicle Dynamics1/3(yd) -> Mux/2, yd/1  "yd"
  Veicle Dynamics1/1(Normal_React) -> Normal_react/1, [Norm_react]
  Veicle Dynamics1/2(xd) -> xd/1, Mux/1  "xd"
  UR5_forces/1 -> Veicle Dynamics1/5(UR5_forces)

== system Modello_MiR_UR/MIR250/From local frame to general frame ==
  Psi : Inport
  Vy : Inport  Port=2
  Vx : Inport  Port=3
  Cos : Trigonometry  Operator=cos
  Product{,1..3} (4 alike) : Product
  Sin : Trigonometry
  Sum : Sum  Inputs=-+
  Sum1 : Sum  Inputs=|++
  Vx_g : Outport
  Vy_g : Outport  Port=2
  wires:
  Product/1 -> Sum/2
  Sin/1 -> Product2/2, Product1/2
  Product1/1 -> Sum/1
  Vx/1 -> Product2/1, Product/1
  Product2/1 -> Sum1/1
  Cos/1 -> Product3/1, Product/2
  Product3/1 -> Sum1/2
  Psi/1 -> Sin/1, Cos/1
  Vy/1 -> Product3/2, Product1/1
  Sum/1 -> Vx_g/1
  Sum1/1 -> Vy_g/1

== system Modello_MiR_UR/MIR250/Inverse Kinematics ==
  vSet : Inport
  psiDotSet : Inport  Port=2
  Demux : Demux  Outputs=2
  MATLAB Function : MATLAB Function  TreatAsAtomicUnit=on
  MATLAB Function1 : MATLAB Function  TreatAsAtomicUnit=on
  Scope1 : Scope
  Scope2 : Scope
  Terminator : Terminator
  ThetaDotL : Outport
  ThetaDotR : Outport  Port=2
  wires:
  vSet/1 -> Demux/1
  Demux/1 -> MATLAB Function1/1(xd_set), MATLAB Function/1(xd_set)  "xd_set"
  psiDotSet/1 -> MATLAB Function1/2(psid_set), MATLAB Function/2(psid_set)
  MATLAB Function/1(Thetad_DR_SET) -> Scope1/1, ThetaDotR/1
  MATLAB Function1/1(Thetad_DL_SET) -> Scope2/1, ThetaDotL/1
  Demux/2 -> Terminator/1  "yd_set"

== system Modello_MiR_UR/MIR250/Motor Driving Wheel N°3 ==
  ThetadL_SET : Inport
  ThetadL_FB : Inport  Port=2
  Gain : Gain  Gain=rap_rid
  Gain1 : Gain  Gain=rap_rid
  Subsystem : Subsystem
  Subsystem1 : Subsystem
  Cm_L : Outport
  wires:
  Subsystem/1(VaRif) -> Subsystem1/1(VaRif)
  Subsystem1/2(iFB) -> Subsystem/3(iFB)
  ThetadL_SET/1 -> Gain1/1
  ThetadL_FB/1 -> Gain/1
  Subsystem1/1(Torque Cm) -> Cm_L/1
  Gain/1 -> Subsystem1/2(Thetad_FB), Subsystem/2(Thetad_FB)
  Gain1/1 -> Subsystem/1(Thetad_SET)

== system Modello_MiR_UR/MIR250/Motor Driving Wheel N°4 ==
  ThetadR_SET : Inport
  ThetadR_FB : Inport  Port=2
  Gain : Gain  Gain=rap_rid
  Gain1 : Gain  Gain=rap_rid
  Subsystem : Subsystem
  Subsystem1 : Subsystem
  Cm_R : Outport
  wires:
  Subsystem1/2(iFB) -> Subsystem/3(iFB)
  ThetadR_SET/1 -> Gain1/1
  Subsystem/1(VaRif) -> Subsystem1/1(VaRif)
  ThetadR_FB/1 -> Gain/1
  Subsystem1/1(Torque Cm) -> Cm_R/1
  Gain/1 -> Subsystem1/2(Thetad_FB), Subsystem/2(Thetad_FB)
  Gain1/1 -> Subsystem/1(Thetad_SET)

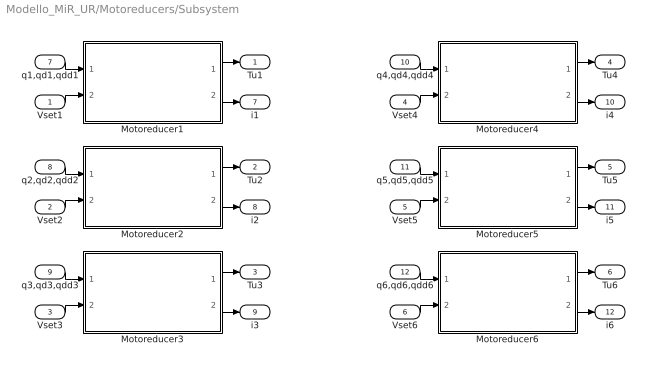
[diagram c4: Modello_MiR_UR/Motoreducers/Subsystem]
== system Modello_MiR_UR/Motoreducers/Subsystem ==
  Vset1 : Inport
  Vset2 : Inport  Port=2
  Vset3 : Inport  Port=3
  Vset4 : Inport  Port=4
  Vset5 : Inport  Port=5
  Vset6 : Inport  Port=6
  q1,qd1,qdd1 : Inport  Port=7
  q2,qd2,qdd2 : Inport  Port=8
  q3,qd3,qdd3 : Inport  Port=9
  q4,qd4,qdd4 : Inport  Port=10
  q5,qd5,qdd5 : Inport  Port=11
  q6,qd6,qdd6 : Inport  Port=12
  Motoreducer1 : Subsystem
  Motoreducer2 : Subsystem
  Motoreducer3 : Subsystem
  Motoreducer4 : Subsystem
  Motoreducer5 : Subsystem
  Motoreducer6 : Subsystem
  Tu1 : Outport
  Tu2 : Outport  Port=2
  Tu3 : Outport  Port=3
  Tu4 : Outport  Port=4
  Tu5 : Outport  Port=5
  Tu6 : Outport  Port=6
  i1 : Outport  Port=7
  i2 : Outport  Port=8
  i3 : Outport  Port=9
  i4 : Outport  Port=10
  i5 : Outport  Port=11
  i6 : Outport  Port=12
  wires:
  Motoreducer5/1(Tu) -> Tu5/1
  q6,qd6,qdd6/1 -> Motoreducer6/1(q,qd,qdd)
  Vset5/1 -> Motoreducer5/2(Vset)
  q5,qd5,qdd5/1 -> Motoreducer5/1(q,qd,qdd)
  Vset1/1 -> Motoreducer1/2(Vset)
  Vset2/1 -> Motoreducer2/2(Vset)
  Vset3/1 -> Motoreducer3/2(Vset)
  q3,qd3,qdd3/1 -> Motoreducer3/1(q,qd,qdd)
  q4,qd4,qdd4/1 -> Motoreducer4/1(q,qd,qdd)
  Motoreducer4/1(Tu) -> Tu4/1
  Vset6/1 -> Motoreducer6/2(Vset)
  Vset4/1 -> Motoreducer4/2(Vset)
  Motoreducer3/1(Tu) -> Tu3/1
  q1,qd1,qdd1/1 -> Motoreducer1/1(q,qd,qdd)
  q2,qd2,qdd2/1 -> Motoreducer2/1(q,qd,qdd)
  Motoreducer6/1(Tu) -> Tu6/1
  Motoreducer2/1(Tu) -> Tu2/1
  Motoreducer1/1(Tu) -> Tu1/1
  Motoreducer1/2(i) -> i1/1
  Motoreducer2/2(i) -> i2/1
  Motoreducer3/2(i) -> i3/1
  Motoreducer4/2(i) -> i4/1
  Motoreducer5/2(i) -> i5/1
  Motoreducer6/2(i) -> i6/1

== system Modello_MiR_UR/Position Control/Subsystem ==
  q1set,qd1set,qdd1set : Inport
  q2set,qd2set,qdd2set : Inport  Port=2
  q3set,qd3set,qdd3set : Inport  Port=3
  q4set,qd4set,qdd4set : Inport  Port=4
  q5set,qd5set,qdd5set : Inport  Port=5
  q6set,qd6set,qdd6set : Inport  Port=6
  q1FB,qd1FB,qdd1FB : Inport  Port=7
  q2FB,qd2FB,qdd2FB : Inport  Port=8
  q3FB,qd3FB,qdd3FB : Inport  Port=9
  q4FB,qd4FB,qdd4FB : Inport  Port=10
  q5FB,qd5FB,qdd5FB : Inport  Port=11
  q6FB,qd6FB,qdd6FB : Inport  Port=12
  Position Control1 : Subsystem
  Position Control2 : Subsystem
  Position Control3 : Subsystem
  Position Control4 : Subsystem
  Position Control5 : Subsystem
  Position Control6 : Subsystem
  Vset1 : Outport
  Vset2 : Outport  Port=2
  Vset3 : Outport  Port=3
  Vset4 : Outport  Port=4
  Vset5 : Outport  Port=5
  Vset6 : Outport  Port=6
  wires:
  q5FB,qd5FB,qdd5FB/1 -> Position Control5/1(qFB,qdFB,qddFB)
  q1FB,qd1FB,qdd1FB/1 -> Position Control1/1(qFB,qdFB,qddFB)
  q6FB,qd6FB,qdd6FB/1 -> Position Control6/1(qFB,qdFB,qddFB)
  q3FB,qd3FB,qdd3FB/1 -> Position Control3/1(qFB,qdFB,qddFB)
  Position Control1/1(Vset) -> Vset1/1
  q4set,qd4set,qdd4set/1 -> Position Control4/2(qset,qdset,qddset)
  Position Control4/1(Vset) -> Vset4/1
  q5set,qd5set,qdd5set/1 -> Position Control5/2(qset,qdset,qddset)
  q1set,qd1set,qdd1set/1 -> Position Control1/2(qset,qdset,qddset)
  q2set,qd2set,qdd2set/1 -> Position Control2/2(qset,qdset,qddset)
  q2FB,qd2FB,qdd2FB/1 -> Position Control2/1(qFB,qdFB,qddFB)
  Position Control5/1(Vset) -> Vset5/1
  Position Control2/1(Vset) -> Vset2/1
  q4FB,qd4FB,qdd4FB/1 -> Position Control4/1(qFB,qdFB,qddFB)
  q6set,qd6set,qdd6set/1 -> Position Control6/2(qset,qdset,qddset)
  Position Control6/1(Vset) -> Vset6/1
  Position Control3/1(Vset) -> Vset3/1
  q3set,qd3set,qdd3set/1 -> Position Control3/2(qset,qdset,qddset)
